INTERFACE I_Count

METHOD M_Count : INT
VAR_INPUT
	bEnable: BOOL;
END_VAR
VAR_OUTPUT
	i_Wert, k_Wert: INT;	
END_VAR
END_METHOD

PROPERTY P_Max_i : INT
GET
END_GET
SET
END_SET
END_PROPERTY

PROPERTY P_Max_k : INT
GET
END_GET
SET
END_SET
END_PROPERTY

END_INTERFACE
